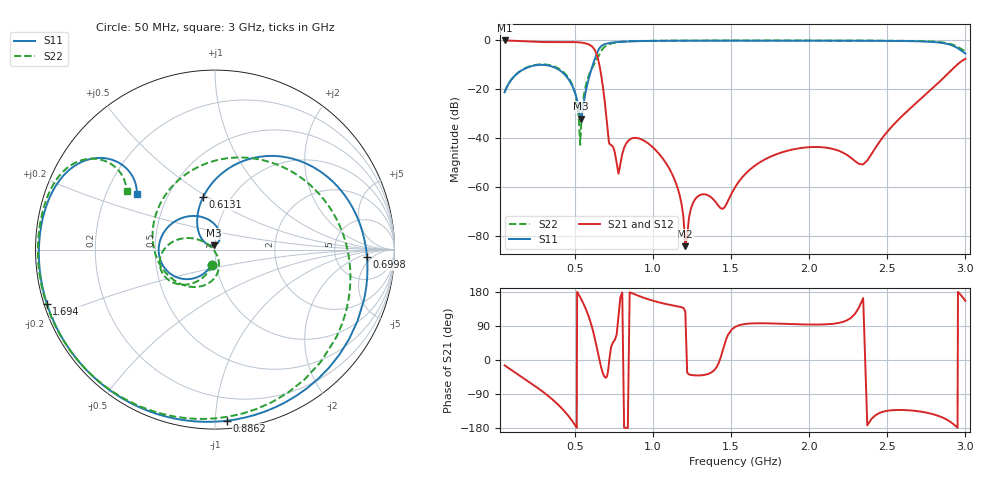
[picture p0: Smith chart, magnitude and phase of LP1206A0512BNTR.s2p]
!	AVX THIN FILM OPERATION
!	LP1206 High Performance Low Pass Filters
!	P/N LP1206A0512BNTR  BN  412134 des D  3 December 2014
# hz S ma R 50
! 2 Port Network Data
! freq  magS11  angS11  magS21  angS21  magS12  angS12  magS22  angS22
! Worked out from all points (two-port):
!   441 points, 50 MHz to 3 GHz, reference 50 ohm
!   highest |S21| = -0.08 dB at 50 MHz (marker M1); lowest = -84.3 dB at 1.207 GHz (marker M2)
!   |S21| within 3 dB of the highest: start of sweep to 617.3 MHz
!   lowest |S11| = -32.0 dB at 538 MHz (marker M3), VSWR 1.05, Z = 49.5 + j2.44 ohm
!   |S11| at or under -10 dB: start of sweep to 615.3 MHz
!   |S22| runs from -42.8 to -0.1 dB; largest |S21 - S12| = 0
!   S11 on the Smith chart (normalised r, x): 50 MHz: 0.95, -0.16; 613.1 MHz: 0.74, +0.48; 699.8 MHz: 11, -3; 886.2 MHz: 0.05, -1.07; 1.694 GHz: 0.01, -0.16; 3 GHz: 0.33, +0.29
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5e7  0.08616 -102.4  0.9905 -14.1  0.9905 -14.1  0.08668 -99.5
1.8475e8  0.2675 -145.7  0.9483 -51.6  0.9483 -51.6  0.271 -133.9
3.820625e8  0.2656 141.2  0.919 -113.7  0.919 -113.7  0.278 178.2
4.83125e8  0.1172 81.8  0.9207 -161.0  0.9207 -161.0  0.1227 150.9
5.38e8  0.02502 100.3  0.898 162.5  0.898 162.5  0.01509 -83.6
5.423333e8  0.0264 118.7  0.8944 159.1  0.8944 159.1  0.02717 -72.9
6.131111e8  0.3004 102.7  0.7255 81.2  0.7255 81.2  0.2836 -142.4
6.583704e8  0.6939 44.3  0.2929 -3.1  0.2929 -3.1  0.5287 76.1
6.997778e8  0.848 -2.8  0.03042 -46.2  0.03042 -46.2  0.7736 -12.9
7.2e8  0.876 -18.7  0.007674 -0.0  0.007674 -0.0  0.8344 -36.1
7.675e8  0.9148 -46.1  0.00306 67.4  0.00306 67.4  0.9075 -69.7
8.8625e8  0.9556 -85.9  0.01005 172.8  0.01005 172.8  0.9616 -108.2
1.040625e9  0.9731 -113.5  0.004657 151.9  0.004657 151.9  0.9783 -131.4
1.206875e9  0.9799 -131.8  6.093e-05 127.6  6.093e-05 127.6  0.9839 -146.2
1.29e9  0.9816 -138.6  0.0006487 -40.7  0.0006487 -40.7  0.9852 -151.7
1.444375e9  0.9833 -149.1  0.000353 22.2  0.000353 22.2  0.9866 -160.1
1.5275e9  0.9837 -153.9  0.001004 87.6  0.001004 87.6  0.9869 -164.0
1.69375e9  0.9839 -162.2  0.003308 97.0  0.003308 97.0  0.9872 -170.8
2.02625e9  0.9823 -176.0  0.006528 93.5  0.006528 93.5  0.9865 177.9
2.345556e9  0.9773 172.1  0.002876 163.4  0.002876 163.4  0.9836 168.2
2.530278e9  0.9698 164.8  0.01728 -132.4  0.01728 -132.4  0.9788 162.3
3e9  0.5351 144.5  0.4156 156.2  0.4156 156.2  0.5903 146.6
